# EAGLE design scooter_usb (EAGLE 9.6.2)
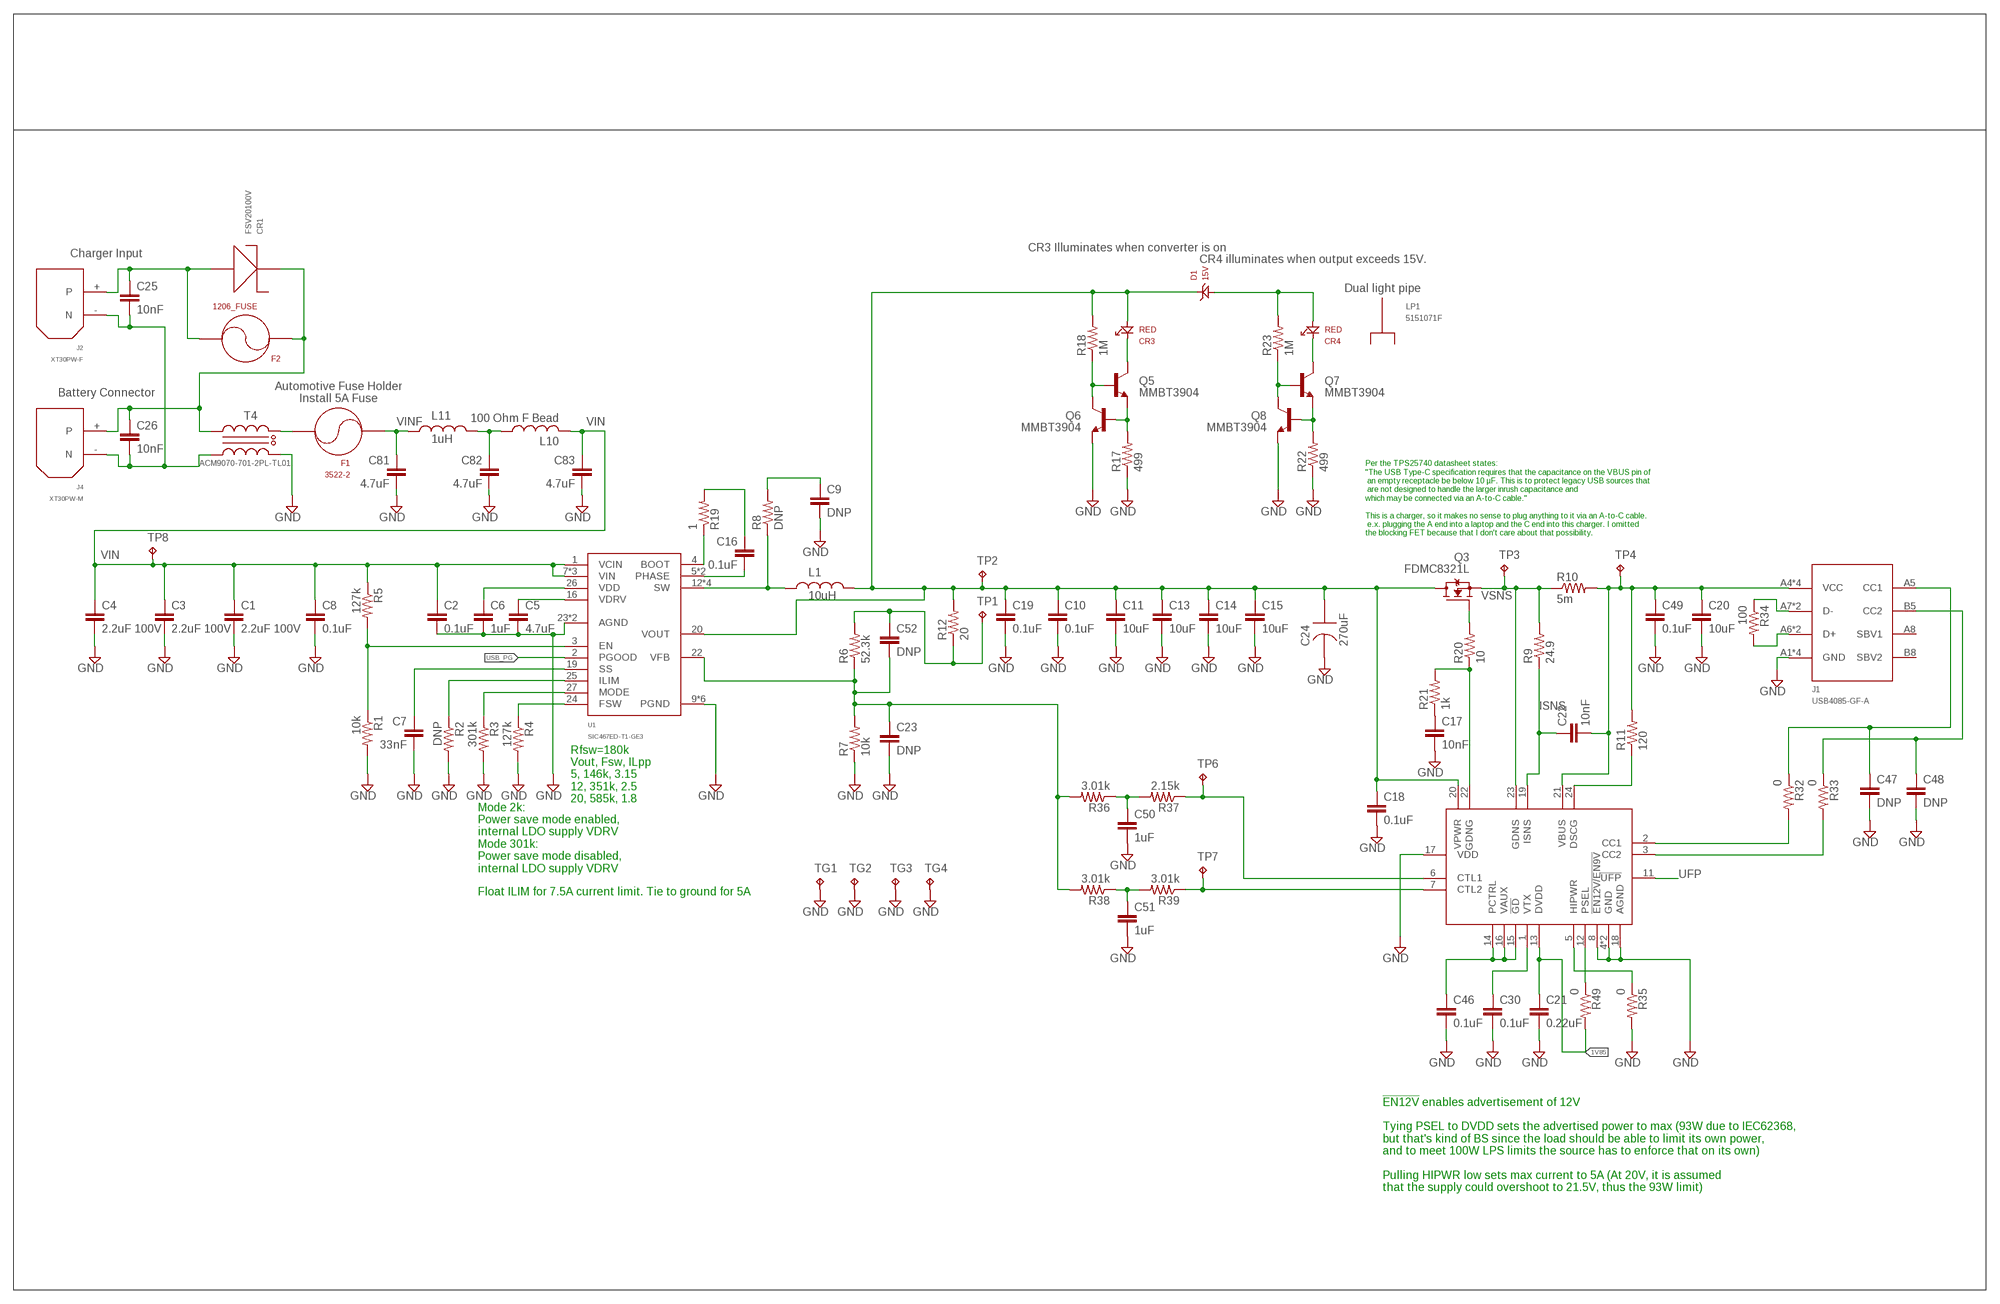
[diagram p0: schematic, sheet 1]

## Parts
C1  2.2uF 100V  C-EUC1210  [C1210]
C2  0.1uF  C-EUC0603  [C0603]
C3  2.2uF 100V  C-EUC1210  [C1210]
C4  2.2uF 100V  C-EUC1210  [C1210]
C5  4.7uF  0805_CAPACITOR  [0805]
C6  1uF  0805_CAPACITOR  [0805]
C7  33nF  C-EUC0603  [C0603]
C8  0.1uF  C-EUC0603  [C0603]
C9  DNP  C-EUC0603  [C0603]
C10  0.1uF  C-EUC0603  [C0603]
C11  10uF  C-EUC1210  [C1210]
C13  10uF  C-EUC1210  [C1210]
C14  10uF  C-EUC1210  [C1210]
C15  10uF  C-EUC1210  [C1210]
C16  0.1uF  0402_CAPACITOR  [0402_INDUCTOR]
C17  10nF  C-EUC0603  [C0603]
C18  0.1uF  C-EUC0603  [C0603]
C19  0.1uF  C-EUC0603  [C0603]
C20  10uF  C-EUC1210  [C1210]
C21  0.22uF  C-EUC0603  [C0603]
C22  10nF  C-EUC0603  [C0603]
C23  DNP  C-EUC0603  [C0603]
C24  270uF  A768MS277M1GLAV022  [A768]
C25  10nF  0805_CAPACITOR  [0805]
C26  10nF  0805_CAPACITOR  [0805]
C30  0.1uF  C-EUC0603  [C0603]
C46  0.1uF  C-EUC0603  [C0603]
C47  DNP  C-EUC0603  [C0603]
C48  DNP  C-EUC0603  [C0603]
C49  0.1uF  C-EUC0603  [C0603]
C50  1uF  C-EUC0603  [C0603]
C51  1uF  C-EUC0603  [C0603]
C52  DNP  C-EUC0603  [C0603]
C81  4.7uF  1210_CAPACITOR  [1210]
C82  4.7uF  1210_CAPACITOR  [1210]
C83  4.7uF  1210_CAPACITOR  [1210]
CR1  FSV20100V  [TO-277]
CR3  RED  150060RS75000  [0603_DIODE]
CR4  RED  150060RS75000  [0603_DIODE]
D1  15V  PDZ15BGWX  [SOD123(AK)]
F1  3522-2  [FUSE_SOCKET]
F2  1206_FUSE  [1206]
J1  USB4085-GF-A  [USBC]
J2  XT30PW-F  [XT30PW-F]
J4  XT30PW-M  [XT30PW-M]
L1  10uH  SRP1265C-100M  [SRP1265]
L10  100 Ohm F Bead  L-USL1812  [L1812]
L11  1uH  NRS8030T1R0NJGJ  [NRS8030]
LP1  5151071F  [5151071F]
Q3  FDMC8321L  [POWER33]
Q5  MMBT3904  MMBT3904-TP  [SOT23-3]
Q6  MMBT3904  MMBT3904-TP  [SOT23-3]
Q7  MMBT3904  MMBT3904-TP  [SOT23-3]
Q8  MMBT3904  MMBT3904-TP  [SOT23-3]
R1  10k  0603_RESISTOR  [0603]
R2  DNP  0603_RESISTOR  [0603]
R3  301k  0603_RESISTOR  [0603]
R4  127k  0603_RESISTOR  [0603]
R5  127k  0603_RESISTOR  [0603]
R6  52.3k  0603_RESISTOR  [0603]
R7  10k  0603_RESISTOR  [0603]
R8  DNP  0603_RESISTOR  [0603]
R9  24.9  0603_RESISTOR  [0603]
R10  5m  1206_RESISTOR  [1206]
R11  120  1206_RESISTOR  [1206]
R12  20  0603_RESISTOR  [0603]
R17  499  0603_RESISTOR  [0603]
R18  1M  0603_RESISTOR  [0603]
R19  1  R-US_R0402  [R0402]
R20  10  0603_RESISTOR  [0603]
R21  1k  0603_RESISTOR  [0603]
R22  499  0603_RESISTOR  [0603]
R23  1M  0603_RESISTOR  [0603]
R32  0  0603_RESISTOR  [0603]
R33  0  0603_RESISTOR  [0603]
R34  100  0603_RESISTOR  [0603]
R35  0  0603_RESISTOR  [0603]
R36  3.01k  0603_RESISTOR  [0603]
R37  2.15k  0603_RESISTOR  [0603]
R38  3.01k  0603_RESISTOR  [0603]
R39  3.01k  0603_RESISTOR  [0603]
R49  0  0603_RESISTOR  [0603]
T4  ACM9070-701-2PL-TL01  [ACM9070]
TG1  TPPAD1-17  [P1-17]
TG2  TPPAD1-17  [P1-17]
TG3  TPPAD1-17  [P1-17]
TG4  TPPAD1-17  [P1-17]
TP1  TPPAD1-17  [P1-17]
TP2  TPPAD1-17  [P1-17]
TP3  TPPAD1-17  [P1-17]
TP4  TPPAD1-17  [P1-17]
TP6  TPPAD1-17  [P1-17]
TP7  TPPAD1-17  [P1-17]
TP8  TPPAD1-17  [P1-17]
U1  SIC467ED-T1-GE3  [MLP55-27L]
U2  TPS25740  [QFN24-44_TI]

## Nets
1V85: C21.1 R49.2 U2.13(DVDD)
20V: Q7.1(B) Q8.3(C) R23.1
BOOT_1: R19.1 U1.4(BOOT)
CC1: R32.2 U2.2(CC1)
CC2: R33.2 U2.3(CC2)
CTL1: R37.1 TP6.TP U2.6(CTL1)
CTL2: R39.1 TP7.TP U2.7(CTL2)
EN_LV: R1.1 R5.2 U1.3(EN)
FB_1: C23.1 C52.2 R6.1 R7.2 R36.2 R38.2 U1.22(VFB)
FSW_1: R4.1 U1.24(FSW)
GND: C1.2 C2.2 C3.2 C4.2 C5.2 C6.2 C7.2 C8.2 C9.2 C10.2 C11.2 C13.2 C14.2 C15.2 C17.2 C18.2 C19.2 C20.2 C21.2 C23.2 C24.- C30.2 C46.2 C47.2 C48.2 C49.2 C50.2 C51.2 C81.2 C82.2 C83.2 J1.A1(GND) J1.A12(GND) J1.B1(GND) J1.B12(GND) Q6.2(E) Q8.2(E) R1.2 R2.2 R3.2 R4.2 R7.1 R17.1 R22.1 R35.2 T4.2IN TG1.TP TG2.TP TG3.TP TG4.TP U1.9(PGND) U1.10(PGND) U1.11(PGND) U1.17(PGND) U1.23(AGND) U1.AGND U1.PGND U1.PGND2(PGND) U2.4(GND) U2.8(!EN12V/EN9V) U2.17(VDD) U2.18(AGND) U2.EP(GND)
ILIM_1: R2.1 U1.25(ILIM)
ISNS: C22.1 R9.1 U2.19(ISNS)
MODE_1: R3.1 U1.27(MODE)
N$1: C9.1 R8.2
N$2: C17.1 R21.1
N$3: Q5.2(E) Q6.1(B) R17.2
N$4: C16.P$1 R19.2
N$5: CR4.A D1.A R23.2
N$6: C52.1 R6.2 R12.1 TP1.TP
N$7: Q3.4(G) R20.2
N$16: R20.1 R21.2 U2.22(GDNG)
N$17: CR3.K Q5.3(C)
N$18: Q7.2(E) Q8.1(B) R22.2
N$19: CR4.K Q7.3(C)
N$33: R11.1 U2.24(DSCG)
N$36: J1.A7(D-) J1.B7(D-) R34.1
N$37: J1.A6(D+) J1.B6(D+) R34.2
N$38: C47.1 J1.A5(CC1) R32.1
N$39: C48.1 J1.B5(CC2) R33.1
N$40: C46.1 U2.14(PCTRL) U2.15(!GD) U2.16(VAUX)
N$43: C30.1 U2.1(VTX)
N$44: R35.1 U2.5(HIPWR)
N$48: C50.1 R36.1 R37.2
N$49: C51.1 R38.1 R39.2
N$63: R49.1 U2.12(PSEL)
ON: Q5.1(B) Q6.3(C) R18.1
P5V1: C10.1 C11.1 C13.1 C14.1 C15.1 C18.1 C19.1 C24.+ CR3.A D1.K L1.P$2 Q3.5(D) Q3.6(D) Q3.7(D) Q3.8(D) Q3.8_P(D) R12.2 R18.2 TP2.TP U1.20(VOUT) U2.20(VPWR)
PHASE_1: C16.P$2 U1.5(PHASE) U1.6(PHASE)
RTN_DIRTY: C25.2 C26.2 J2.-(N) J4.-(N) T4.2OUT
SS_1: C7.1 U1.19(SS)
SW_1: L1.P$1 R8.1 U1.12(SW) U1.13(SW) U1.14(SW) U1.SW
UFP: U2.11(!UFP)
USB_PG: U1.2(PGOOD)
VCHGIN: C25.1 CR1.1 CR1.2 F2.2 J2.+(P)
VDD_1: C6.1 U1.26(VDD)
VDRV_1: C5.1 U1.16(VDRV)
VF5: C82.1 L10.1 L11.P$2
VIN: C1.1 C2.1 C3.1 C4.1 C8.1 C83.1 L10.2 R5.1 TP8.TP U1.1(VCIN) U1.7(VIN) U1.8(VIN) U1.VIN
VIN_DIRTY: C26.1 CR1.3 F2.1 J4.+(P) T4.1OUT
VINF: C81.1 F1.1A F1.2A L11.P$1
VINN: F1.3B F1.4B T4.1IN
VSNS: Q3.1(S) Q3.2(S) Q3.3(S) R9.2 R10.1 TP3.TP U2.23(GDNS)
VUSB: C20.1 C22.2 C49.1 J1.A4(VCC) J1.A9(VCC) J1.B4(VCC) J1.B9(VCC) R10.2 R11.2 TP4.TP U2.21(VBUS)
Unconnected: J1.A8(SBV1) J1.B8(SBV2)

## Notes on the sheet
- CR3 Illuminates when converter is on
- Charger Input
- CR4 illuminates when output exceeds 15V.
- Dual light pipe
- Battery Connector
- Automotive Fuse Holder
  Install 5A Fuse
- Per the TPS25740 datasheet states: 
  "The USB Type-C specification requires that the capacitance on the VBUS pin of
   an empty receptacle be below 10 µF. This is to protect legacy USB sources that
   are not designed to handle the larger inrush capacitance and
  which may be connected via an A-to-C cable."
  
  This is a charger, so it makes no sense to plug anything to it via an A-to-C cable.
   e.x. plugging the A end into a laptop and the C end into this charger. I omitted
  the blocking FET because that I don't care about that possibility.
- Rfsw=180k
  Vout, Fsw, ILpp
  5, 146k, 3.15
  12, 351k, 2.5
  20, 585k, 1.8
- Mode 2k:
  Power save mode enabled, 
  internal LDO supply VDRV
  Mode 301k:
  Power save mode disabled, 
  internal LDO supply VDRV
- Float ILIM for 7.5A current limit. Tie to ground for 5A
- !EN12V! enables advertisement of 12V
  
  Tying PSEL to DVDD sets the advertised power to max (93W due to IEC62368, 
  but that's kind of BS since the load should be able to limit its own power, 
  and to meet 100W LPS limits the source has to enforce that on its own)
  
  Pulling HIPWR low sets max current to 5A (At 20V, it is assumed
  that the supply could overshoot to 21.5V, thus the 93W limit)

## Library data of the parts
C1 C3 C4 C11 C13-C15 C20 = rcl:C-EU: CAPACITOR, European symbol; PARTNO: 490-11659-1-ND
C2 C7-C10 C17-C19 C21-C23 C30 C46-C52 = rcl:C-EU: CAPACITOR, European symbol; PARTNO: NA; SPICEPREFIX: C
C5 C6 C25 C26 = ruark2:0805_CAPACITOR: NO DEFINED PN
C16 = ruark2:0402_CAPACITOR: 0402 select capacitor; VALUE: sel
C24 = ruark2:A768MS277M1GLAV022: 270 µF 40 V Aluminum - Polymer Capacitors Radial, Can - SMD 22mOhm 2000 Hrs @ 125°C; PARTNO: 399-A768MS277M1GLAV022CT-ND
C81-C83 = ruark2:1210_CAPACITOR: NO VALUE
CR1 = ruark2:FSV20100V: Diode Schottky 100V 20A Surface Mount TO-277-3; PARTNO: FSV20100VCT-ND
CR3 CR4 = ruark2:150060RS75000: Red 625nm LED Indication - Discrete 2V 0603 (1608 Metric); PARTNO: 732-4978-1-ND
D1 = ruark2:PDZ15BGWX: Zener Diode 15V 365mW ±2.13% Surface Mount SOD-123; PARTNO: 1727-7703-1-ND
F1 = ruark2:3522-2: FUSE CLIP BLADE 500V 20A PCB; PARTNO: 36-3522-2-ND
F2 = ruark2:1206_FUSE
J1 = ruark2:USB4085-GF-A: USB - C USB 2.0 Receptacle Connector 16 Position Through Hole, Right Angle; PARTNO: 2073-USB4085-GF-ACT-ND
J2 = ruark2:XT30PW-F
J4 = ruark2:XT30PW-M
L1 = ruark2:SRP1265C-100M: 10µH Shielded Wirewound Inductor 12A 18mOhm Max Nonstandard; PARTNO: SRP1265A-220MCT-ND
L10 = rcl:L-US: INDUCTOR, American symbol; SPICEPREFIX: L
L11 = ruark2:NRS8030T1R0NJGJ: 1µH Shielded Wirewound Inductor 6.2A 11.7mOhm Max Nonstandard; PARTNO: 587-2962-1-ND
LP1 = ruark2:5151071F: Light Pipe 2 Wide Clear Rigid Round with Flat Top, 3mm Board Mount, Press Fit; PARTNO: 350-1590-ND
Q3 = ruark2:FDMC8321L: N-Channel 40 V 22A (Ta), 49A (Tc) 2.3W (Ta), 40W (Tc) Surface Mount Power33; PARTNO: FDMC8321LCT-ND
Q5-Q8 = ruark2:MMBT3904-TP: Bipolar (BJT) Transistor NPN 40V 200mA 300MHz 350mW Surface Mount SOT-23 (SMD 2N3904); PARTNO: MMBT3904TPMSCT-ND
R1-R9 R12 R17 R18 R20-R23 R32-R39 R49 = ruark2:0603_RESISTOR: 0603 Resistor -- WARNING: NO DEFINED PART NUMBER OR VALUE; VALUE: sel
R10 R11 = ruark2:1206_RESISTOR: NO DEFINED PN; VALUE: sel
R19 = rcl:R-US_: RESISTOR, American symbol; SPICEPREFIX: R
T4 = ruark2:ACM9070-701-2PL-TL01: 2 Line Common Mode Choke Surface Mount 700 Ohms @ 100MHz 5A DCR 10mOhm; PARTNO: 445-2216-1-ND
TG1-TG4 TP1-TP4 TP6-TP8 = testpad:TP: Test pad
U1 = ruark2:SIC467ED-T1-GE3: Buck Switching Regulator IC Positive Adjustable 0.8V 1 Output 6A PowerPAK® MLP55-27 60V; PARTNO: SIC467ED-T1-GE3CT-ND
U2 = ruark2:TPS25740: USB, Type-C Controller PMIC 24-VQFN (4x4); PARTNO: 296-44487-1-ND

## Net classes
1 HV: clearance 0.406 mm

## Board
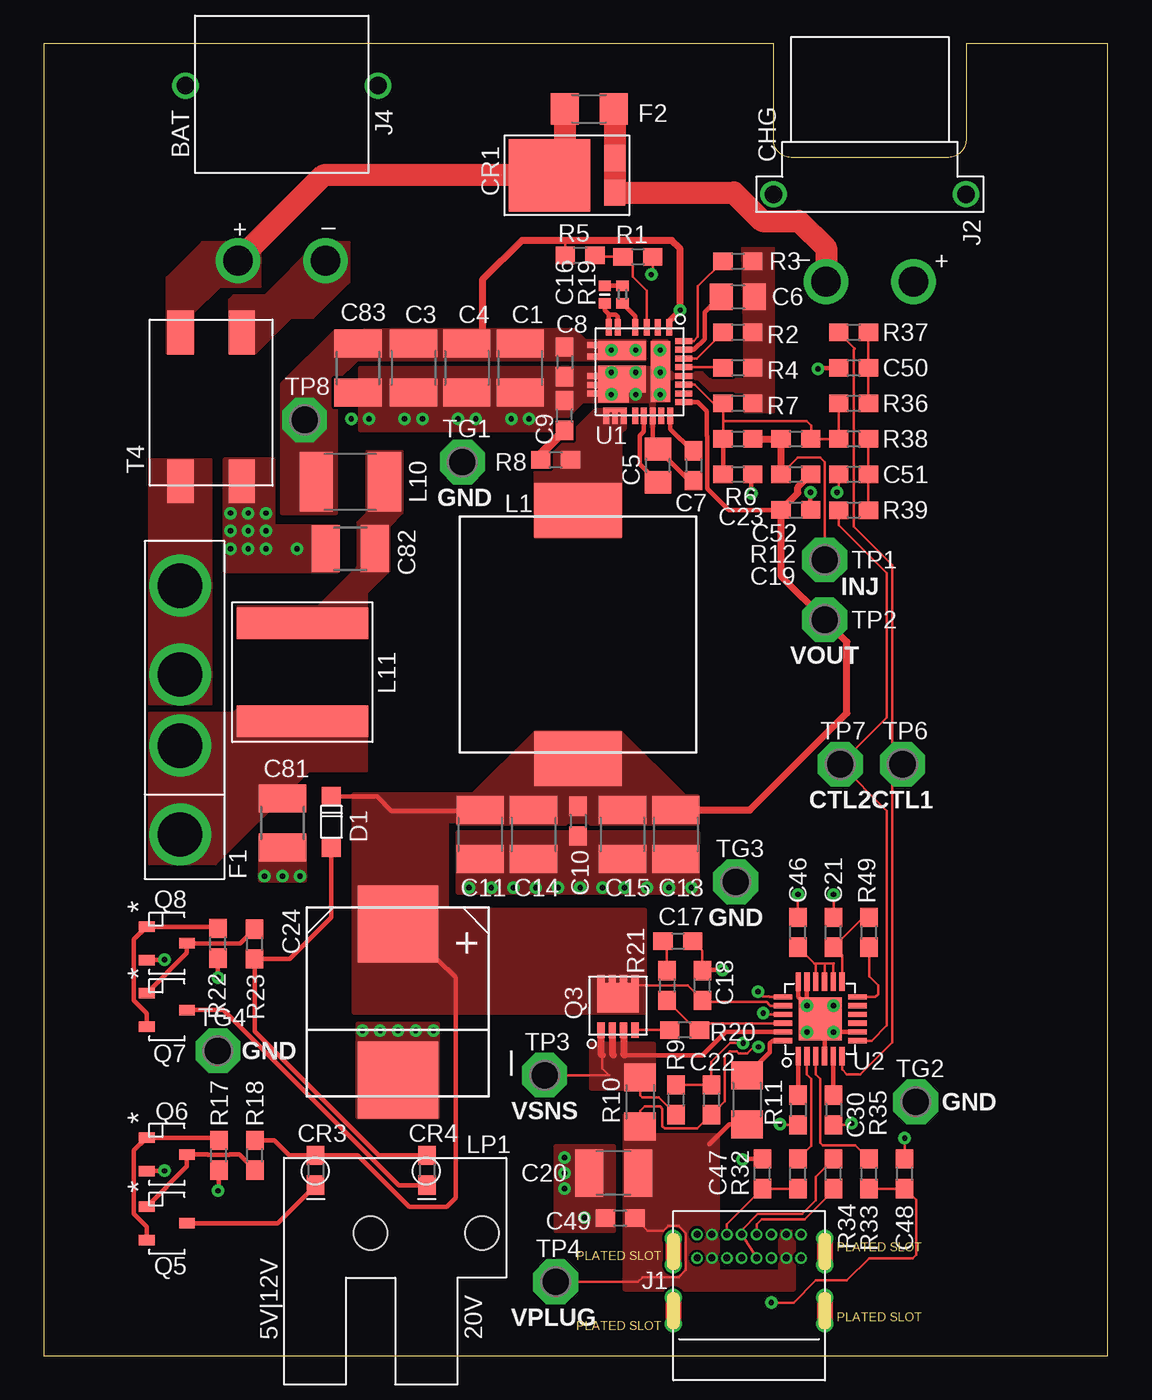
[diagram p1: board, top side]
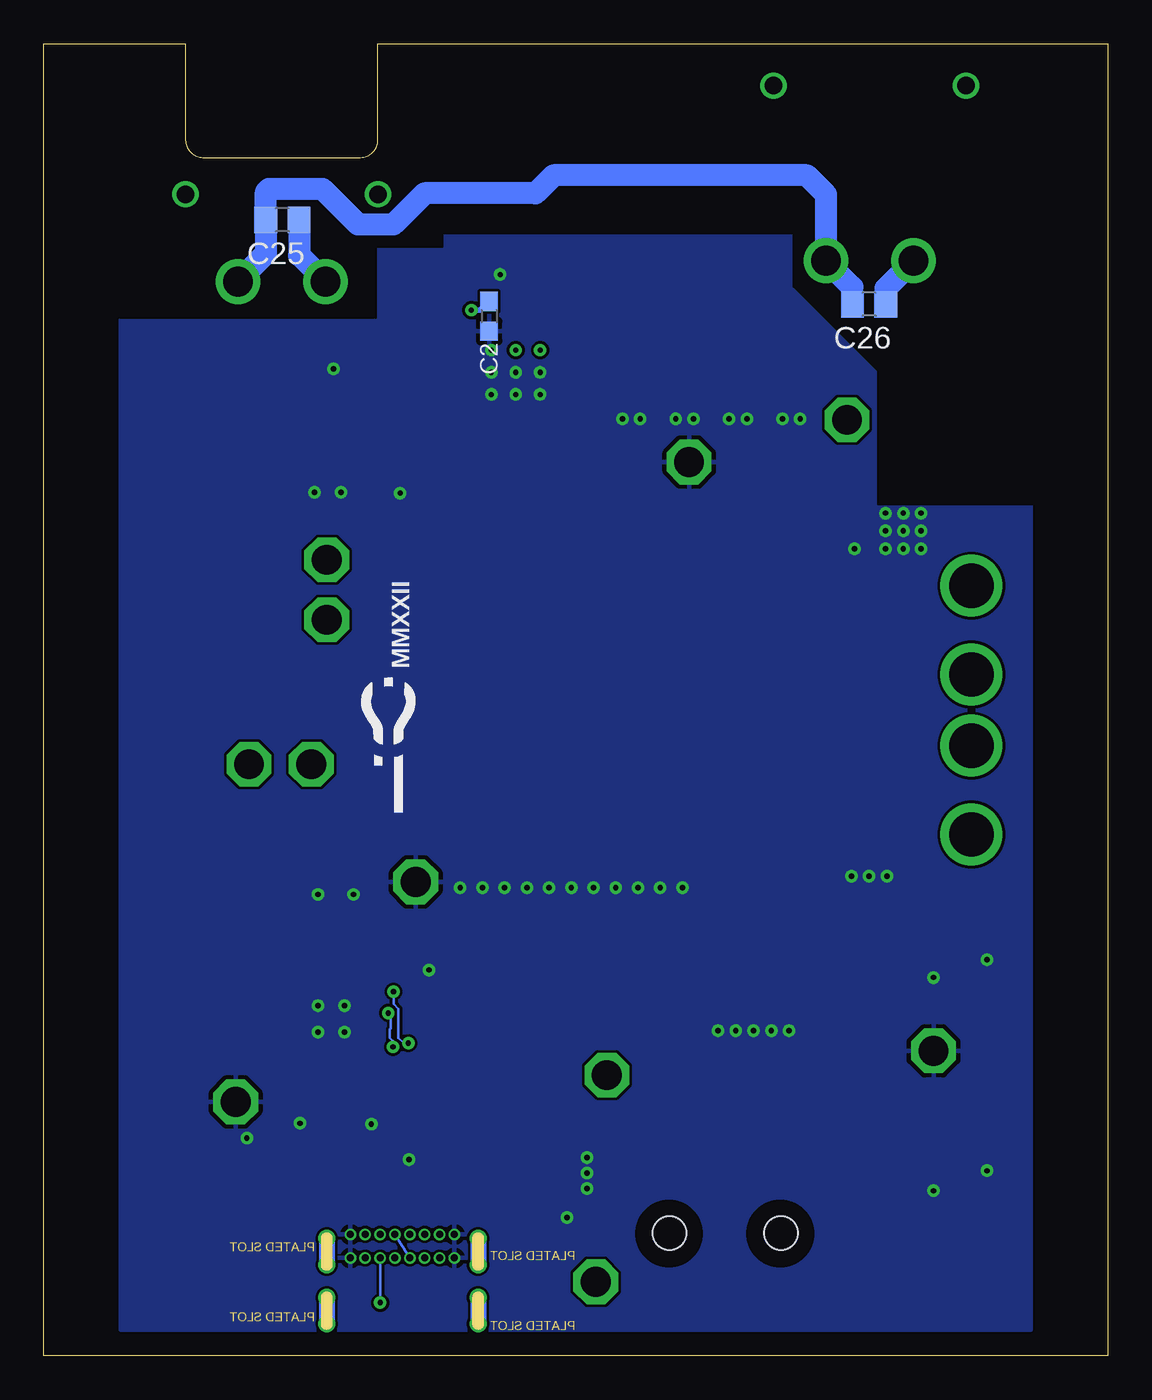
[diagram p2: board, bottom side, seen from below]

Size 60.8 x 75 mm. Coordinates in mm from the lower left corner, seen from the top.
Outline: 0,0 60.8,0 60.8,75 52.7,75 52.7,69.5 arc-90 51.7,68.5 42.7,68.5 arc-90 41.7,69.5 41.7,75 0,75 0,0
Copper layers (1*16): Top 0.035mm / dielectric 1.5mm / Bottom 0.035mm
Design rules "default *": minimum track width 6mil, minimum drill 12mil, track to track 6mil, track to pad 6mil, pad to pad 6mil, via to via 6mil, smd to smd 6mil, copper to edge 0mil, drill to drill 6mil, minimum pad ring 0.13mm, minimum via ring 8mil, stop-mask expansion 4mil, vias tented up to drill 12mil, thermal gap 10mil
bRestrict: area 1.4,48.7 to 18,73.3; area 17.7,59.3 to 59.4,73.3; area 16.9,5.2 to 20.5,8.8; area 23.3,5.2 to 26.8,8.8

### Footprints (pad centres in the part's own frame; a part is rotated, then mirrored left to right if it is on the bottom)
C1210 = smd 1.6 x 2.7: 1 -1.4,0; 2 1.4,0
C0603 = smd 1.1 x 1: 1 -0.85,0; 2 0.85,0
0805 = smd 1.3 x 1.5: 1 -0.95,0; 2 0.95,0
0402_INDUCTOR = smd 0.6 x 0.7: P$1 0.5,0; P$2 -0.5,0
A768 = smd 4.4 x 4.6: + -4.45,0; - 4.45,0
1210 = smd 1.6 x 2.7: 1 -1.4,0; 2 1.4,0
TO-277 = smd 1.2 x 1.5: 1 2.75,0.985; 2 2.75,-0.985 | smd 4.65 x 4.15: 3 -1,0
0603_DIODE = smd 1.1 x 1: A -0.85,0; K 0.85,0
SOD123(AK) = smd 1.1 x 1.1: A 1.45,0; K -1.45,0
FUSE_SOCKET = drill 2.54: 1A -7.112,0; 2A -2.032,0; 3B 2.032,0; 4B 7.112,0
1206 = smd 1.6 x 1.8: 1 -1.4,0; 2 1.4,0
USBC = drill 0.4 pad 0.65: A1 -2.975,0.98; A4 -2.125,0.98; A5 -1.275,0.98; A6 -0.425,0.98; A7 0.425,0.98; A8 1.275,0.98; A9 2.125,0.98; A12 2.975,0.98; B1 2.975,-0.37; B4 2.125,-0.37; B5 1.275,-0.37; B6 0.425,-0.37; B7 -0.425,-0.37; B8 -1.275,-0.37; B9 -2.125,-0.37; B12 -2.975,-0.37 | drill 0.65 pad 0.9: P$1 -4.325,0.75; P$2 4.325,0.75; P$3 4.325,-0.75; P$4 -4.325,-2.63; P$5 -4.325,-0.75; P$6 -4.325,-4.13; P$7 4.325,-2.63; P$8 4.325,-4.13
XT30PW-F = drill 1.7: + -2.5,0; - 2.5,0 | drill 1: P$3 5.5,5; P$4 -5.5,5
XT30PW-M = drill 1.7: + -2.5,-14; - 2.5,-14 | drill 1: P$3 5.5,-4; P$4 -5.5,-4
SRP1265 = smd 3.1 x 5: P$1 -7.1,0; P$2 7.1,0
L1812 = smd 1.9 x 3.4: 1 -1.95,0; 2 1.95,0
NRS8030 = smd 1.8 x 7.5: P$1 -2.8,0; P$2 2.8,0
5151071F = hole 1.93: -3.175,0; 3.175,0
POWER33 = smd 0.42 x 0.9: 1 -0.975,-1.4; 2 -0.325,-1.4; 3 0.325,-1.4; 4 0.975,-1.4; 5 0.975,1.3; 6 0.325,1.3; 7 -0.325,1.3; 8 -0.975,1.3 | smd 2.37 x 1.7: 8_P 0,0.45
SOT23-3 = smd 0.6 x 0.9: 1 0.32,-1.15; 2 2.22,-1.15; 3 1.27,1.15
0603 = smd 1.1 x 1: 1 -0.85,0; 2 0.85,0
R0402 = smd 0.6 x 0.7: 1 -0.5,0; 2 0.5,0
ACM9070 = smd 2.5 x 1.5: 1IN -4.25,1.75; 1OUT 4.25,1.75; 2IN -4.25,-1.75; 2OUT 4.25,-1.75
P1-17 = drill 1.702 pad 2.54 octagon: TP 0,0
MLP55-27L = smd 0.95 x 0.34: 1 -0.025,4.207; 2 -0.025,3.555; 3 -0.025,2.902; 4 -0.025,2.25; 5 -0.025,1.25; 6 -0.025,0.75; 12 5.025,0.6; 13 5.025,1.1; 14 5.025,1.6; 15 5.025,2.25; 16 5.025,2.75; 17 5.025,3.25; 18 5.025,3.75; 19 5.025,4.25 | smd 0.34 x 0.95: 7 0.98,-0.025; 8 1.63,-0.025; 9 2.76,-0.025; 10 3.26,-0.025; 11 3.76,-0.025; 20 4.25,5.025; 21 3.75,5.025; 22 3.25,5.025; 23 2.75,5.025; 24 2.25,5.025; 25 1.75,5.025; 26 1.25,5.025; 27 0.75,5.025 | smd 3.5 x 1.1: AGND 2.5,3.7 | smd 0.58 x 1.73: PGND 3.98,1.02 | smd 1.52 x 2.7: PGND2 2.93,1.5 | smd 0.25 x 1: SW 4.675,1.1 | smd 1.1 x 2.7: VIN 1.3,1.5
QFN24-44_TI = smd 1.05 x 0.3: 1 -2.125,1.25; 2 -2.125,0.75; 3 -2.125,0.25; 4 -2.125,-0.25; 5 -2.125,-0.75; 6 -2.125,-1.25; 13 2.125,-1.25; 14 2.125,-0.75; 15 2.125,-0.25; 16 2.125,0.25; 17 2.125,0.75; 18 2.125,1.25 | smd 0.3 x 1.05: 7 -1.25,-2.125; 8 -0.75,-2.125; 9 -0.25,-2.125; 10 0.25,-2.125; 11 0.75,-2.125; 12 1.25,-2.125; 19 1.25,2.125; 20 0.75,2.125; 21 0.25,2.125; 22 -0.25,2.125; 23 -0.75,2.125; 24 -1.25,2.125 | smd 2.45 x 2.45: EP 0,0

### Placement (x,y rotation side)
C1  27.22,56.47 270 top
C2  35.35,59.42 270 bottom
C3  21.13,56.47 270 top
C4  24.18,56.47 270 top
C5  35.1,50.88 90 top
C6  39.67,60.53 0 top
C7  37.13,50.88 270 top
C8  29.76,56.8 270 top
C9  29.76,53.76 90 top
C10  30.53,30.56 270 top
C11  24.94,29.8 270 top
C13  36.11,29.8 270 top
C14  27.99,29.8 270 top
C15  33.07,29.8 270 top
C16  32.05,60.66 90 top
C17  36.24,23.7 0 top
C18  37.64,21.16 90 top
C19  42.97,48.35 0 top
C20  32.56,10.45 180 top
C21  45.13,24.21 90 top
C22  38.15,14.64 270 top
C23  39.67,50.38 0 top
C24  20.24,20.23 270 top
C25  47.16,64.93 180 bottom
C26  13.64,60.11 180 bottom
C30  43.1,14.05 270 top
C46  43.1,24.21 90 top
C47  41.07,10.4 90 top
C48  49.2,10.4 90 top
C49  32.94,7.86 180 top
C50  46.27,56.47 180 top
C51  46.27,50.37 180 top
C52  42.97,52.41 0 top
C81  13.64,30.47 270 top
C82  17.53,46.14 180 top
C83  17.95,56.47 270 top
CR1  29.89,67.47 0 top
CR3  15.54,10.6 270 top
CR4  21.89,10.6 270 top
D1  16.43,30.52 270 top
F1  7.79,36.91 90 top
F2  31.16,71.28 0 top
J1  40.31,5.96 0 top
J2  47.2,61.4 0 top
J4  13.6,76.6 0 top
L1  30.53,41.23 270 top
L10  17.53,49.95 180 top
L11  14.78,39.08 90 top
LP1  21.86,7 0 top
Q3  32.81,20.02 0 top
Q5  7.03,8.84 270 top
Q6  7.03,12.78 270 top
Q7  7.03,21.04 270 top
Q8  7.03,24.85 270 top
R1  33.96,62.82 0 top
R2  39.67,58.5 0 top
R3  39.67,62.57 0 top
R4  39.67,56.47 0 top
R5  30.65,62.9 0 top
R6  39.67,52.41 0 top
R7  39.67,54.44 180 top
R8  29.26,51.22 180 top
R9  36.11,14.64 270 top
R10  34.08,14.51 270 top
R11  40.18,14.64 270 top
R12  42.97,50.38 0 top
R17  10,11.46 90 top
R18  12.06,11.46 90 top
R19  33.07,60.66 90 top
R20  36.62,18.62 180 top
R21  35.61,21.16 270 top
R22  9.95,23.58 90 top
R23  12.03,23.53 270 top
R32  43.1,10.4 90 top
R33  47.16,10.4 90 top
R34  45.13,10.4 90 top
R35  45.13,14.05 270 top
R36  46.27,54.44 180 top
R37  46.27,58.5 0 top
R38  46.27,52.41 180 top
R39  46.27,48.34 0 top
R49  47.16,24.21 90 top
T4  9.56,54.24 90 top
TG1  23.92,51.09 0 top
TG2  49.83,14.51 0 top
TG3  39.54,27.09 0 top
TG4  9.95,17.43 0 top
TP1  44.62,45.5 270 top
TP2  44.62,42.07 0 top
TP3  28.62,16.04 0 top
TP4  29.26,4.23 0 top
TP6  49.07,33.82 0 top
TP7  45.51,33.82 0 top
TP8  14.91,53.5 0 top
U1  31.54,58.76 270 top
U2  44.37,19.26 90 top

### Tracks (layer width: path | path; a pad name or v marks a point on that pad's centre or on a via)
1V85
  Top 0.152: U2.13 45.62,22.87 C21.1 46.83,25.06 R49.2
20V
  Top 0.254: Q7.1 8.18,23.02 Q8.3 11.23,23.58 R23.1
BOOT_1
  Top 0.254: U1.4 33.79,59.44 R19.1
CC1
  Top 0.152: R32.2 43.86,12.01 43.86,15.83 43.61,16.08 43.61,17.12 U2.2
CC2
  Top 0.152: R33.2 46.38,12.03 44.52,12.03 44.37,12.18 44.37,15.83 44.12,16.08 U2.3
CTL1
  Top 0.152: U2.6 45.62,16.36 45.89,16.08 46.66,16.08 48.47,17.9 | 48.47,17.9 48.48,17.91 | R37.1 46.35,57.58 46.27,57.51 46.27,47.41 48.48,45.2 48.48,34.4 TP6.TP 48.47,33.22 48.47,31.29 48.48,31.28 48.48,18.75 48.47,18.74 48.47,17.9
CTL2
  Top 0.152: U2.7 47.31,18.01 48.18,18.88 48.18,31.15 TP7.TP 48.18,36.48 48.18,43.09 48.18,43.34 48.18,44.74 45.42,47.49 R39.1 45.39,48.3
EN_LV
  Top 0.152: U1.3 34.45,60.88 33.65,61.68 33.65,62.27 R1.1 31.58,62.82 R5.2
FB_1
  Top 0.152: U1.22 37.21,55.51 38.27,54.44 R7.2 38.82,53.42 | R6.1 38.82,53.42 | C52.2 43.86,52.41 | 43.86,52.41 R38.2 R36.2 | 43.86,52.41 43.86,53.17 43.61,53.42 38.82,53.42
  Top 0.254: C23.1 R6.1
FSW_1
  Top 0.152: U1.24 38.78,56.51 R4.1
GND  (via drill 0.3)
  Top 0.152: 38.74,22.01 v38.78,22.05 | R35.2 45.93,13.2 v46.15,13.29 | C48.2 v49.2,12.43 | C46.2 v43.1,26.37 | C21.2 v45.13,26.37 | C17.2 37.64,23.16 37.64,22.05 | R1.2 34.81,61.89 v34.72,61.8 | C30.2 42.12,13.2 v42.08,13.24 | C51.2 45.42,49.45 v45.34,49.36
  Top 0.254: U1.17 34.79,52.14 C5.2 36.9,50.03 C7.2 | U2.4 44.62,18.5 v43.61,18.5 | U2.EP 44.37,18.5 v45.13,18.5 v45.13,18.51 U2.8 | U2.17 43.61,21.38 v43.61,20.02 43.12,20.51 U2.18 | C18.2 37.64,22.05 v38.78,22.05 | C50.2 44.29,56.47 v44.24,56.42 | C23.2 40.43,50.29 v40.43,49.31 | R22.1 v9.95,21.62 | Q8.2 6.89,22.63 v6.9,22.64 | Q6.2 5.9,10.58 v6.9,10.58 | R17.1 10,9.61 v9.95,9.43 | C47.2 39.97,11.25 v39.92,11.21 | C19.2 v43.81,49.36
  other vias: 32.43,56.22 32.43,54.95 33.83,56.22 35.23,57.49 35.23,56.22 35.23,54.95 20.62,53.55 21.64,53.55 23.67,53.55 24.68,53.55 26.72,53.55 27.73,53.55 45.13,20.02 14.48,46.14 13.64,27.42 14.65,27.42 12.62,27.42 24.3,26.75 25.57,26.75 26.84,26.75 28.11,26.75 29.38,26.75 30.65,26.75 31.92,26.75 33.19,26.75 34.46,26.75 35.73,26.75 37,26.75 18.59,53.55 17.57,53.55 10.67,48.17 11.68,48.17 10.67,47.15 11.68,47.15 12.7,48.17 12.7,47.15 10.67,46.14 11.68,46.14 12.7,46.14 29.76,10.45 29.76,11.34 29.76,9.56 30.91,7.91 33.83,54.95 18.21,18.58 19.22,18.58 20.24,18.58 21.26,18.58 22.27,18.58
  pour Bottom: 4.4,73.06 56.4,73.06 56.4,1.5 4.4,1.5
  pour Top (no thermals): 35.48,55.84 37.38,55.84 38.15,55.07 40.05,55.07 40.05,53.93 41.7,53.93 41.7,63.33 39.92,63.33 40.05,55.84 38.02,55.84 37.64,56.22 35.48,56.22
  pour Top (no thermals): 18.08,52.91 18.08,56.47 34.84,56.47 34.84,57.99 35.61,57.99 35.61,54.69 34.84,54.69 34.84,53.17 34.72,53.17 34.72,54.56 30.78,54.56 29.13,52.91
  pour Top (no thermals): 23.67,26.5 23.67,29.93 37.38,29.93 37.38,26.5
  pour Top (no thermals): 16.76,44.87 16.76,47.41 13.13,47.41 13.13,51.22 10.33,51.22 10.33,44.87
  pour Top (no thermals): 14.91,29.71 12.37,29.71 12.37,27.17 14.91,27.17
  pour Top (no thermals): 32.56,7.15 32.56,11.97 29.26,11.97 29.26,7.15
  pour Top (no thermals): 17.95,13.62 22.53,13.62 22.53,18.96 17.95,18.96
ILIM_1
  Top 0.152: U1.25 37.32,57.01 R2.1
ISNS  (via drill 0.3)
  Top 0.152: R9.1 C22.1 38.15,16.8 39.22,17.87 v39.97,17.87 | v40.81,20.81 41.09,20.53 41.44,20.53 41.46,20.51 U2.19
  Bottom 0.152: v40.81,20.81 40.81,20.12 40.53,19.84 40.53,18.17 40.24,17.87 v39.97,17.87
MODE_1
  Top 0.152: U1.27 37.14,58.01 37.38,58.25 37.38,61.13 R3.1
N$1
  Top 0.508: R8.2 28.41,51.55 C9.1
N$2
  Top 0.152: R21.1 35.61,23.49 C17.1
N$3
  Top 0.254: Q5.2 5.88,7.38 5.15,8.11 5.15,11.73 Q6.1 9.85,12.46 R17.2
N$4
  Top 0.254: C16.P$1 R19.2
N$5
  Top 0.254: D1.A 16.43,25.05 14.06,22.68 R23.2 12.07,22.64 12.07,18.54 19.16,11.45 CR4.A
N$6
  Top 0.152: R12.1 43.09,51.34 44.37,51.34 44.62,51.09 TP1.TP
  Top 0.406: R6.2 C52.1 R12.1
N$7
  Top 0.152: R20.2 Q3.4
N$16
  Top 0.152: U2.22 37.86,19.01 R20.1 37.3,18.62 R21.2
N$17
  Top 0.254: CR3.K 13.36,7.57 Q5.3
N$18
  Top 0.254: R22.2 9.85,24.53 Q8.1 5.15,23.8 5.15,20.3 5.88,19.57 Q7.2
N$19
  Top 0.254: Q7.3 10.26,19.77 20.28,9.75 CR4.K
N$33
  Top 0.254: U2.24 41.64,18.01 41.48,17.85 41.48,17.34 R11.1
N$36
  Top 0.152: J1.A7 40.73,7.52 41.02,7.81 43.48,7.81 45.13,9.46 R34.1
  Bottom 0.152: J1.B7 J1.A7
N$37
  Top 0.152: J1.B6 J1.A6 39.88,7.18 40.81,8.12 43.35,8.12 44.12,8.88 44.12,10.24 R34.2
N$38
  Top 0.152: R32.1 C47.1 39.03,7.52 J1.A5
N$39  (via drill 0.3)
  Top 0.152: R33.1 C48.1 49.85,8.9 49.85,5.76 49.66,5.58 47.16,5.58 45.89,4.31 44.12,4.31 42.85,3.04 v41.58,3.04
  Bottom 0.152: J1.B5 v41.58,3.04
N$40
  Top 0.152: U2.16 44.12,22.43 | U2.15 44.62,22.43 | 44.62,22.43 44.12,22.43 | U2.14 45.12,22.42 45.13,22.43 | 45.13,22.43 | 45.13,22.43 44.62,22.43 | 44.12,22.43 44.03,22.43 C46.1
N$43
  Top 0.254: U2.1 43.12,14.92 C30.1
N$44
  Top 0.254: U2.5 45.12,14.91 R35.1
N$48
  Top 0.152: R36.1 C50.1 R37.2
N$49
  Top 0.152: R39.2 C51.1 R38.1
N$63
  Top 0.152: R49.1 47.16,21.67 47.67,21.16 47.67,20.66 47.52,20.51 U2.12
ON
  Top 0.254: Q5.1 8.18,10.82 Q6.3 9.36,11.51 9.38,11.49 10.62,11.49 10.64,11.51 11.17,11.51 R18.1
P5V1
  Top 0.152: 37.94,20.01 37.73,20.22 | 37.73,20.22 C18.1 36.79,21.16 33.95,21.16 Q3.5 | U2.20 41.52,20.01 41.31,20.22 37.73,20.22 | C13.1 37.39,31.2
  Top 0.254: 22.53,22.64 23.54,21.62 23.54,9.03 23.03,8.52 20.88,8.52 17.95,11.45 CR3.A 14.03,11.45 13.17,12.32 R18.2 | U1.20 37.38,54.52 37.89,54.01 37.89,52.56 37.91,52.56 37.91,49.56 39.13,48.35 C19.1 | D1.K 19.04,31.96 19.86,31.15 24.89,31.15 C11.1
  Top 0.406: C13.1 40.36,31.2 45.89,36.74 45.89,40.8 TP2.TP 42.12,44.57 C19.1 | 42.16,48.35 C19.1 | C19.1 43.1,49.32 43.1,49.66 43.52,50.07 R12.2
  pour Top (no thermals): 28.11,35.64 24.43,31.96 23.67,31.96 23.67,30.43 37.38,30.43 37.38,31.96 36.62,31.96 32.94,35.64
  pour Top (no thermals): 26.34,30.56 26.34,32.09 17.7,32.09 17.7,19.64 34.34,19.64 34.34,25.48 23.03,25.48 23.03,30.56
PHASE_1
  Top 0.254: U1.5 32.79,59.41 32.69,59.52 32.3,59.52 | 32.3,59.52 32.29,59.51 U1.6 | 32.3,59.52 32.05,59.77 C16.P$2
RTN_DIRTY
  Bottom 1.27: C26.2 14.59,61.09 J4.- 16.1,66.38 17.19,67.47 31.67,67.47 32.69,66.46 39.04,66.46 40.81,64.68 42.85,64.68 44.88,66.71 47.93,66.71 48.11,66.52 C25.2 48.11,62.99 J2.-
  pour Top (no thermals): 10.59,57.31 10.59,60.36 10.84,60.61 12.62,60.61 15.67,63.66 17.45,63.66 17.45,61.38 15.41,59.34 14.14,59.34 12.11,57.31
SS_1
  Top 0.254: U1.19 35.79,52.98 37.04,51.73 C7.1
SW_1
  Top 0.254: 30.54,48.34 L1.P$1
  pour Top (no thermals): 32.94,46.82 32.94,52.79 33.19,53.04 33.19,54.06 31.54,54.06 28.11,50.63 28.11,46.82
VCHGIN
  Top 1.27: F2.2 32.64,71.2 CR1.1 CR1.2 39.44,66.49 41.06,64.86 43.17,64.86 44.7,63.33 J2.+
  Bottom 1.27: J2.+ 46.21,62.91 C25.1
VDD_1
  Top 0.254: U1.26 37.15,57.51 37.77,58.12 37.77,59.64 38.66,60.53 C6.1
VDRV_1
  Top 0.254: U1.16 34.29,52.82 34.07,52.6 34.07,50.96 C5.1
VF5
  pour Top (no thermals): 11.1,41.06 18.46,41.06 18.46,43.6 19.73,44.87 19.73,47.41 20.49,48.17 20.49,51.72 18.46,51.72 18.46,48.17 17.95,47.66 17.95,45.12 15.67,42.83 11.1,42.83
VIN  (via drill 0.3)
  Top 0.152: 29.8,57.69 C8.1 | R5.1 29.8,63.67 29.89,63.76
  Top 0.305: U1.1 35.75,59.15 v36.37,59.77
  Top 0.406: v36.37,59.77 36.37,63.28 35.89,63.76 29.89,63.76 27.32,63.76 25.07,61.5 25.07,57.82
  Bottom 0.305: C2.1 35.85,59.77 v36.37,59.77
  other vias: 32.43,57.49 33.83,57.49
  pour Top (no thermals): 19.86,58.63 16.68,58.58 13.64,55.53 13.64,48.17 16.68,48.17 16.68,55.79 17.87,56.98 34.34,56.98 34.34,57.99 30.91,57.99 30.27,58.63
VIN_DIRTY
  Top 1.27: J4.+ 15.97,67.47 CR1.3 29.76,68.34 F2.1
  Bottom 1.27: C26.1 12.69,61.01 J4.+
  pour Top (no thermals): 8.56,57.31 8.56,59.6 10.08,61.12 12.37,61.12 12.37,63.66 9.06,63.66 7.03,61.63 7.03,57.31
VINF
  pour Top (no thermals): 6.02,28.1 6.02,36.74 10.84,36.74 11.1,36.99 18.46,36.99 18.46,33.44 15.16,33.44 9.83,28.1
VINN
  pour Top (no thermals): 6.02,51.22 9.06,51.22 9.57,51.22 9.57,37.25 6.02,37.25
VSNS
  Top 0.152: R10.1 34.08,14.89 34.21,14.77 35.14,14.77 R9.2 | TP3.TP 32.3,16.04 31.92,16.42 31.92,17.18
  Top 0.254: U2.23 38.97,18.51 37.64,17.18 33.19,17.18 | 33.19,18.57 Q3.3
  Top 0.406: Q3.1 31.84,17.27 31.92,17.18 | Q3.2 32.49,17.25 32.56,17.18 | Q3.3 33.14,17.24 33.19,17.18
  pour Top (no thermals): 34.84,15.27 34.84,17.82 31.29,17.82 31.29,15.27
VUSB  (via drill 0.3)
  Top 0.152: U2.21 41.2,19.51 v41.11,19.59 | R10.2 34.08,14 34.34,14.26 35.21,14.26 35.35,14.12 35.35,13.12 35.48,12.99 37.35,12.99 C22.2 38.91,14.55 38.91,17.13 39.19,17.41 39.61,17.41 39.73,17.29 40.21,17.29 40.58,17.66 v40.85,17.66 | TP4.TP 33.96,4.23 34.22,4.49 36.28,4.49 36.7,4.91 36.7,7 36.28,7.42 35.68,7.42 35.41,7.15 34.5,7.15 C49.1
  Top 0.254: R11.2 39.16,13.24 38.02,12.1
  Bottom 0.152: v41.11,19.59 40.97,19.45 40.97,18.71 41.02,18.67 41.02,18.18 40.85,18.01 v40.85,17.66
  pour Top (no thermals): 33.19,3.8 42.85,3.8 42.85,7.1 42.08,7.1 42.08,4.81 38.53,4.81 38.53,12.61 34.84,12.61 34.84,13.75 33.19,13.75

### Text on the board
tPlace: BAT | CHG | GND | INJ | VOUT | CTL2 | CTL1 | GND | GND | GND | VSNS | VPLUG | 5V|12V | 20V
bPlace: MMXXII
bStop: 033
